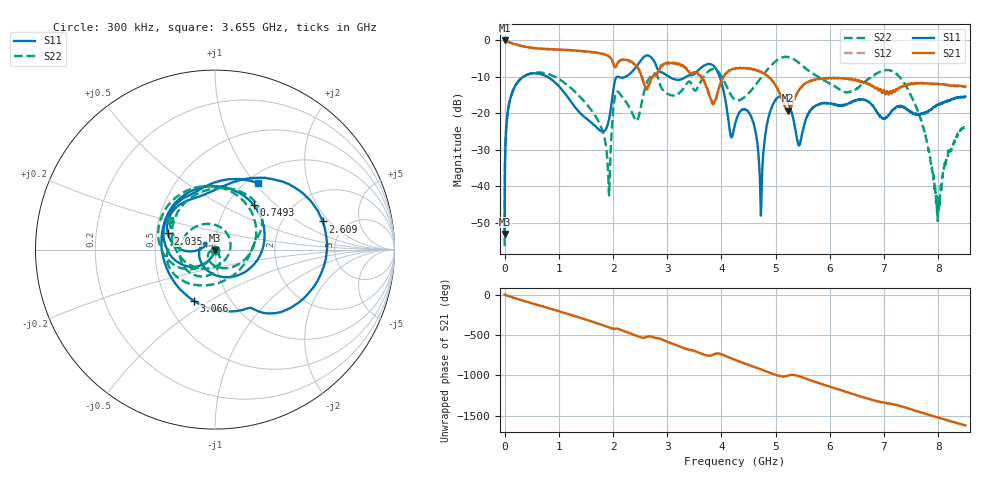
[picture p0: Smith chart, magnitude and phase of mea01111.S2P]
!Agilent Technologies,E5071B,MY42402595,A.08.01
!Date: Tue Jan 02 09:42:42 2001
!Data & Calibration Information:
!Freq	S11:SOLT2(ON)	S21:SOLT2(ON)	S12:SOLT2(ON)	S22:SOLT2(ON)
# Hz S dB R 50
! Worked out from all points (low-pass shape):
!   1601 points, 300 kHz to 8.5 GHz, reference 50 ohm
!   highest |S21| = 0.00 dB at 300 kHz (marker M1); lowest = -19.2 dB at 5.233 GHz (marker M2)
!   |S21| within 3 dB of the highest: start of sweep to 1.501 GHz
!   lowest |S11| = -53.0 dB at 300 kHz (marker M3), VSWR 1.00, Z = 50 - j0.223 ohm
!   |S11| at or under -10 dB: start of sweep to 339.6 MHz; 791.1 MHz to 2.068 GHz (1.276 GHz wide, 89.3 % of centre); 3.969 GHz to end of sweep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
!   |S22| runs from -56.4 to -4.4 dB; largest |S21 - S12| = 0.027
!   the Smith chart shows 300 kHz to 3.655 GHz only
!   S11 on the Smith chart (normalised r, x): 300 kHz: 1.00, -0.00; 749.3 MHz: 1.32, +0.73; 2.035 GHz: 0.58, +0.11; 2.609 GHz: 3.33, +1.70; 3.066 GHz: 0.68, -0.43; 3.655 GHz: 1.12, +1.03
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300000  -53.04 -91.5  -0.00 0.0  0.01 0.0  -56.42 -114.3
5.342312e7  -20.13 -127.2  -0.34 -14.3  -0.35 -14.4  -20.16 -124.6
1.331078e8  -14.59 -150.8  -0.76 -32.6  -0.79 -32.6  -14.63 -143.7
7.493361e8  -9.67 49.1  -2.32 -156.6  -2.37 -156.3  -8.98 94.4
1.418687e9  -20.25 -153.8  -2.91 67.4  -2.89 67.0  -15.86 -27.6
1.912732e9  -22.51 174.6  -4.24 -42.3  -4.22 -42.4  -37.37 -155.9
2.034916e9  -11.11 161.1  -7.21 -63.5  -7.31 -63.1  -15.39 -118.0
2.608645e9  -4.15 14.6  -13.19 -169.3  -13.43 -167.0  -12.23 166.1
2.837075e9  -8.25 -57.7  -8.45 180.0  -8.62 177.2  -10.65 26.9
3.065504e9  -10.21 -112.5  -6.19 118.7  -5.90 118.4  -15.01 -37.7
3.655171e9  -7.13 57.3  -10.80 -16.3  -10.49 -17.0  -10.39 146.3
4.25015e9  -23.03 -16.4  -7.69 -87.7  -7.69 -87.9  -16.23 29.9
4.537015e9  -20.50 -64.0  -7.76 -158.9  -7.73 -159.6  -13.88 37.0
4.728258e9  -48.03 -26.9  -8.52 153.6  -8.61 153.5  -10.29 20.9
4.914189e9  -18.82 16.8  -10.60 106.3  -10.57 106.6  -6.91 -10.3
5.232928e9  -17.27 -86.3  -19.24 77.8  -19.19 76.9  -4.59 -89.1
5.429483e9  -28.65 139.0  -13.65 69.8  -13.68 69.5  -6.10 -138.2
5.668537e9  -18.78 9.3  -10.93 13.4  -11.02 13.8  -8.90 179.1
7.086925e9  -20.39 -83.6  -14.82 91.7  -14.31 89.7  -8.15 31.0
7.644718e9  -20.34 -106.4  -11.72 -12.0  -11.77 -11.4  -20.02 -75.7
7.990018e9  -17.56 -108.1  -11.94 -80.7  -11.87 -81.3  -49.53 -175.1
8.5e9  -15.36 -134.7  -12.69 -180.0  -12.68 178.9  -23.94 59.1
